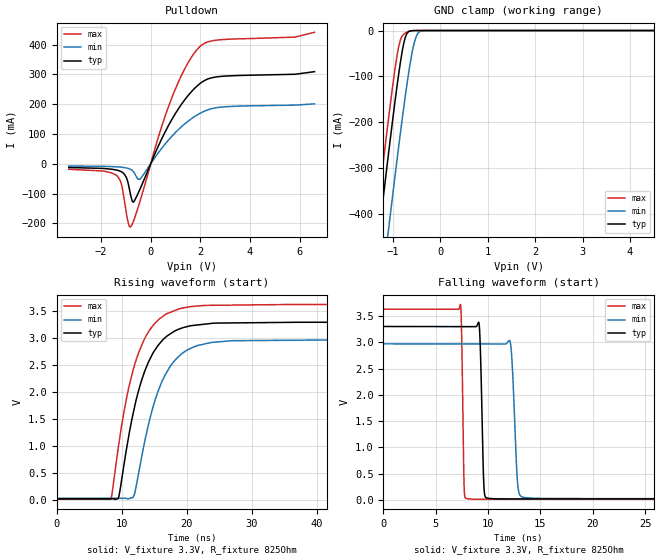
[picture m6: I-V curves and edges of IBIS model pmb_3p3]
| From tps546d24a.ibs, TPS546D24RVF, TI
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|   pmb_3p3 Model
[Model]   pmb_3p3
Model_type   I/O_open_drain
Polarity   Inverting
Enable   Active-High
Vinl = 0.8
Vinh = 1.35
Vmeas = 1.65
Vref = 3.3
Cref = 2pF
Rref = 825
|   typ   min   max
C_comp   3.204pF   3.154pF   3.248pF
|C_comp_pull_down   3.764pF   3.578pF   4.184pF
|  Where Nom  PVT is Nominal Process, 3.3V,   25C
|   Fast PVT is Strong Process,  3.63V, -40C
|   Slow PVT is Weak Process,   2.97V, 150C
[Voltage Range]   3.3   2.97   3.63
|Junction Temperature
[Temperature Range]   25   150   -40
[Pullup Reference]   3.3   2.97   3.63
[Pulldown Reference]   0   0   0
[Power Clamp Reference]   3.3   2.97   3.63
[GND Clamp Reference]   0   0   0
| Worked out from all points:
|   slope of the pulldown table from 0 to 0.495 V, typ, clamps not added: 5.36 ohm
|   GND clamp passes 1 mA (typ) near -0.63 V on its own axis
|   falling waveform, V_fixture 3.3V, R_fixture 825Ohm: 20-80 % time 233ps typ, 371ps min, 165ps max; typ from 3.3 V to 0.02 V
|   rising waveform, V_fixture 3.3V, R_fixture 825Ohm: 20-80 % time 4.08ns typ, 4.19ns min, 3.99ns max; typ from 0.02 V to 3.3 V
[Pulldown]
|   Voltage   I(typ)   I(min)   I(max)
-3.3V     -12.66mA   -7.595mA   -18.68mA
-1.36V    -21.58mA   -10.54mA   -40.68mA
-1.171V   -27.5mA    -11.8mA    -71.96mA
-983.4mV  -46.01mA   -14.19mA   -165.1mA
-815.1mV  -104mA     -18.99mA   -212.9mA
-706.2mV  -128.8mA   -25.95mA   -195.3mA
-438.9mV  -86.31mA   -52.3mA    -127.7mA
848.1mV   148.1mA    91.9mA     221mA
1.432V    221.3mA    138mA      328.1mA
1.957V    267.3mA    167.8mA    391.3mA
2.788V    292.6mA    189.6mA    415.9mA
6.6V      308.9mA    200.9mA    440.9mA
[GND Clamp]
|   Voltage   I(typ)   I(min)   I(max)
-3.3V     -2.303A    -2.451A    -2.239A
-1.488V   -619mA     -784.4mA   -542.6mA
-1.31V    -458.9mA   -625.3mA   -381.7mA
-1.241V   -397.5mA   -564.1mA   -320.2mA
-1.112V   -285.2mA   -451.4mA   -208.6mA
-1.053V   -234.6mA   -400.1mA   -159.1mA
-874.5mV  -92.54mA   -250.1mA   -33.68mA
-775.5mV  -30.4mA    -171.2mA   -8.346mA
-696.3mV  -5.423mA   -112.3mA   -3.045mA
-537.9mV  -83.47uA   -22.2mA    -96.93uA
-399.3mV  -1.542uA   -973.9uA   -950.8nA
6.6V      0A         0A         0A
[POWER Clamp]
|   Voltage   I(typ)   I(min)   I(max)
-3.3V     0A         0A         0A
0V        0A         0A         0A
6.6V      0A         0A         0A
[Ramp]
R_load = 825
|   typ   min   max
dV/dt_r   1.96829/4.06354e-09   1.76496/4.16569e-09   2.16942/3.97337e-09
dV/dt_f   1.96829/2.33392e-10   1.76496/3.70671e-10   2.16942/1.65038e-10
[Falling Waveform]
V_fixture = 3.3V
V_fixture_min = 2.97V
V_fixture_max = 3.63V
R_fixture = 825Ohm
C_fixture = 0F
|   Time   V(typ)   V(min)   V(max)
0s        3.3V       2.97V      3.63V
7.357ns   3.298V     2.968V     3.718V
7.734ns   3.298V     2.968V     144.3mV
8.545ns   3.297V     2.968V     16.8mV
9.182ns   3.245V     2.968V     16.79mV
9.652ns   128.5mV    2.968V     16.79mV
10.73ns   22.73mV    2.968V     16.78mV
12.09ns   22.73mV    3.021V     16.78mV
14.44ns   22.71mV    33.65mV    16.77mV
500ns     19.51mV    28.39mV    14.29mV
[Rising Waveform]
V_fixture = 3.3V
V_fixture_min = 2.97V
V_fixture_max = 3.63V
R_fixture = 825Ohm
C_fixture = 0F
|   Time   V(typ)   V(min)   V(max)
0s        19.51mV    28.39mV    14.29mV
8.34ns    20.19mV    28.89mV    10.77mV
9.58ns    60.65mV    28.96mV    1.039V
11.74ns   1.584V     43.2mV     2.395V
13.57ns   2.395V     1.091V     3.001V
14.84ns   2.729V     1.73V      3.241V
16.23ns   2.958V     2.204V     3.4V
19.21ns   3.19V      2.711V     3.559V
22.48ns   3.261V     2.889V     3.611V
500ns     3.3V       2.97V      3.63V
